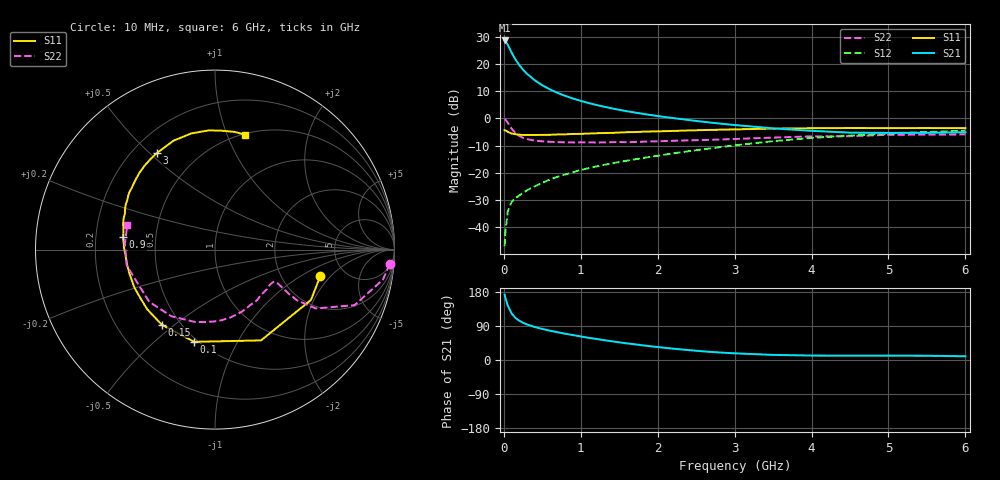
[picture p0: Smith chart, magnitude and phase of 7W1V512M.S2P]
! Infineon Technologies  Discrete & RF Semiconductors
! BFS17W
! Si NPN RF Bipolar Junction Transistor in SOT323
! VCE = 1.5 V  IC = 12 mA
! Common Emitter S-Parameters:  August  1999
# GHz  S  MA  R  50
!  f  S11  S21  S12  S22
! GHz  MAG  ANG  MAG  ANG  MAG  ANG  MAG  ANG
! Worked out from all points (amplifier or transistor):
!   36 points, 10 MHz to 6 GHz, reference 50 ohm
!   highest |S21| = 28.6 dB at 10 MHz (marker M1)
!   |S21| within 3 dB of that: start of sweep to 75.68 MHz
!   unconditionally stable (mu >= 1): 331.4 MHz to end of sweep
!   at 250 MHz: K = 0.89, MSG = 22.6 dB, |S12| = -27.3 dB
!   at 1.4 GHz: K = 1.26, MAG = 7.0 dB, |S12| = -16.6 dB
!   at 6 GHz: K = 1.10, MAG = -2.2 dB, |S12| = -4.5 dB
!   S11 on the Smith chart (normalised r, x): 10 MHz: 3.31, -1.52; 100 MHz: 0.48, -0.68; 150 MHz: 0.40, -0.45; 900 MHz: 0.32, +0.06; 3 GHz: 0.30, +0.53; 6 GHz: 0.51, +1.16
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0.01  0.6051 -13.9  26.99 172.5  0.0045 84.9  0.9764 -4.7
0.02  0.6039 -27.7  26.49 164.2  0.0082 80.5  0.951 -10.1
0.05  0.5672 -63.1  22.65 144.2  0.0191 65.7  0.837 -21.7
0.1  0.5268 -102.7  16.26 123.3  0.0291 54.0  0.65 -30.3
0.15  0.5128 -125.4  12.13 111.2  0.0345 51.4  0.538 -31.7
0.2  0.5032 -138.7  9.559 103.7  0.0385 53.2  0.4778 -30.9
0.25  0.4954 -148.4  7.818 98.1  0.043 52.4  0.4389 -29.7
0.3  0.4963 -155.1  6.607 93.9  0.0477 55.2  0.4178 -29.0
0.4  0.4955 -164.9  5.035 87.1  0.0563 58.4  0.39 -28.1
0.5  0.4973 -171.3  4.06 81.9  0.0654 60.5  0.3789 -28.2
0.6  0.4994 -176.3  3.397 77.3  0.0755 61.7  0.3716 -29.0
0.7  0.5064 179.3  2.937 73.2  0.0848 62.9  0.3664 -30.8
0.9  0.5172 172.4  2.311 65.7  0.1031 64.3  0.361 -35.0
1.1  0.5265 166.1  1.917 58.6  0.1218 64.2  0.3617 -40.4
1.3  0.5388 160.5  1.641 52.4  0.1403 64.3  0.3614 -46.7
1.6  0.5576 153.0  1.353 43.9  0.167 64.3  0.3656 -56.2
2.2  0.5883 139.0  1.013 29.9  0.2271 63.4  0.3877 -77.2
3  0.6277 121.0  0.755 17.6  0.3195 58.6  0.4183 -105.4
3.5  0.6493 110.8  0.656 13.5  0.3818 53.7  0.444 -123.2
4.5  0.6653 93.0  0.547 11.4  0.4811 41.1  0.4709 -157.0
5.5  0.6649 80.4  0.543 11.2  0.5615 29.3  0.5033 176.1
6  0.661 75.6  0.557 9.8  0.5936 23.6  0.5076 164.2
